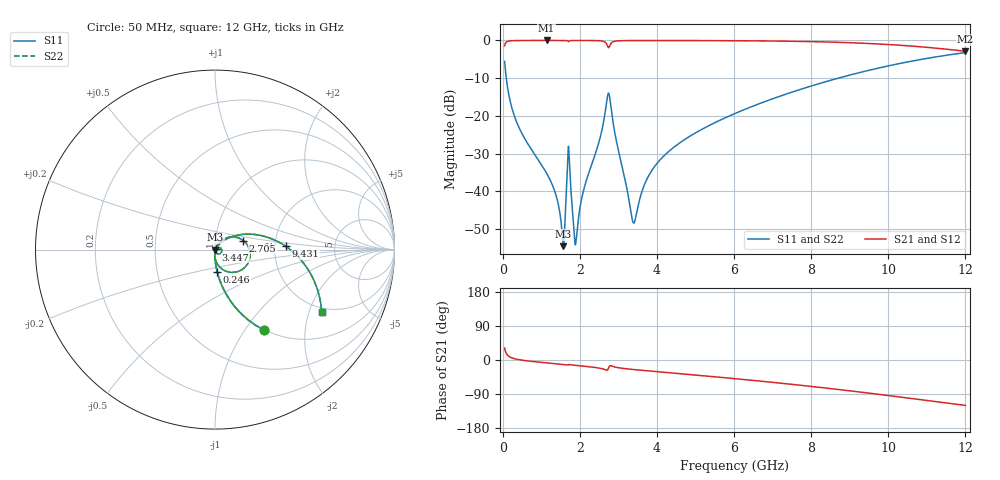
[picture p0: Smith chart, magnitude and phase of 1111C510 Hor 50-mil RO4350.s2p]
# GHz S MA R 50
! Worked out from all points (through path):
!   11951 points, 50 MHz to 12 GHz, reference 50 ohm
!   highest |S21| = -0.01 dB at 1.139 GHz (marker M1); lowest = -2.9 dB at 12 GHz (marker M2)
!   group delay of S21, straight-line fit = 28.1 ps
!   lowest |S11| = -54.5 dB at 1.575 GHz (marker M3), VSWR 1.00, Z = 50.2 - j0.0674 ohm
!   |S11| at or under -10 dB: 92.99 MHz to 8.705 GHz (8.612 GHz wide, 196 % of centre)
!   |S22| runs from -54.5 to -3.2 dB; largest |S21 - S12| = 0
!   S11 on the Smith chart (normalised r, x): 50 MHz: 0.99, -1.24; 246 MHz: 0.99, -0.25; 2.705 GHz: 1.37, +0.14; 3.447 GHz: 1.01, +0.00; 9.431 GHz: 2.30, +0.10; 12 GHz: 1.84, -2.44
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0.05  0.5275 -58.5  0.8493 31.5  0.8493 31.5  0.5275 -58.5
0.246  0.1235 -84.5  0.9918 5.2  0.9918 5.2  0.1235 -84.5
1.139  0.01738 -94.1  0.9987 -7.6  0.9987 -7.6  0.01738 -94.1
1.385  0.008807 -91.9  0.9987 -9.9  0.9987 -9.9  0.008807 -91.9
1.575  0.001874 -21.0  0.9981 -11.8  0.9981 -11.8  0.001874 -21.0
1.707  0.03948 -19.1  0.9607 -12.6  0.9607 -12.6  0.03948 -19.1
1.745  0.01667 -74.5  0.992 -12.2  0.992 -12.2  0.01667 -74.5
1.831  0.003895 -68.0  0.9976 -13.5  0.9976 -13.5  0.003895 -68.0
1.879  0.001977 -20.2  0.9979 -14.1  0.9979 -14.1  0.001977 -20.2
2.042  0.007717 59.6  0.9979 -15.7  0.9979 -15.7  0.007717 59.6
2.522  0.05021 57.4  0.9891 -21.6  0.9891 -21.6  0.05021 57.4
2.705  0.1656 17.7  0.875 -26.8  0.875 -26.8  0.1656 17.7
2.782  0.1662 -49.6  0.8581 -15.4  0.8581 -15.4  0.1662 -49.6
3.352  0.004422 -50.2  0.9958 -24.7  0.9958 -24.7  0.004422 -50.2
3.447  0.004449 11.0  0.9962 -25.7  0.9962 -25.7  0.004449 11.0
3.683  0.01249 48.1  0.9967 -27.9  0.9967 -27.9  0.01249 48.1
4.034  0.02451 52.5  0.9967 -31.1  0.9967 -31.1  0.02451 52.5
6.025  0.1076 39.1  0.9909 -49.3  0.9909 -49.3  0.1076 39.1
8.017  0.2502 19.2  0.9638 -69.9  0.9638 -69.9  0.2502 19.2
9.431  0.3942 2.7  0.9137 -86.6  0.9137 -86.6  0.3942 2.7
10.009  0.4606 -4.5  0.8819 -93.9  0.8819 -93.9  0.4606 -4.5
12  0.689 -30.4  0.7178 -119.8  0.7178 -119.8  0.689 -30.4
